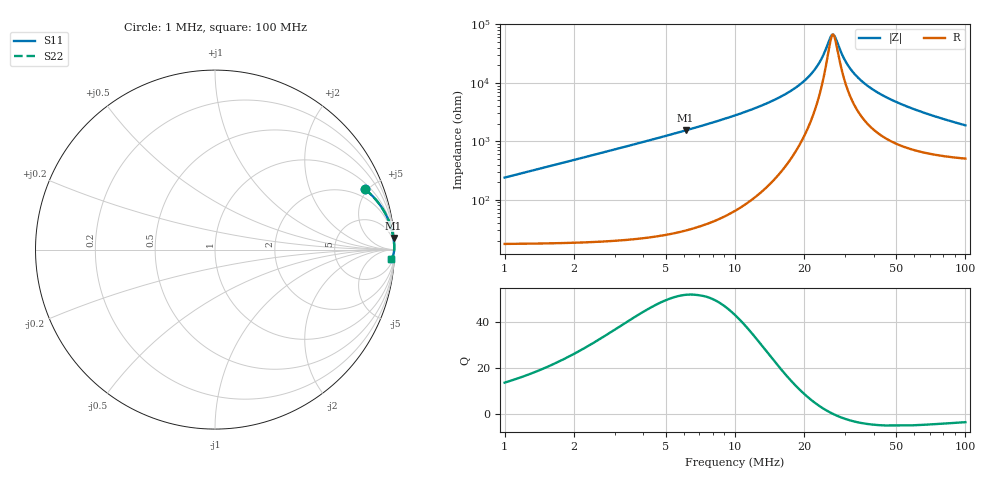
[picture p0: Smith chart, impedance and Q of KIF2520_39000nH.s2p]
!version-2
!date-12.2020
!Series
# MHz S RI R 50
!Freq ReS11 ImS11 ReS21 ImS21 ReS12 ImS12 ReS22 ImS22
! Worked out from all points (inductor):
!   991 points, 1 MHz to 100 MHz, reference 50 ohm
!   read as one part in series: L = 37.9 uH near 1.4 MHz
!   highest Q = 51.7 at 6.1 MHz (marker M1), where L = 40 uH
!   self-resonance near 26.6 MHz
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1  0.8339 0.3373  0.1661 -0.3373  0.1661 -0.3373  0.8339 0.3373
1.9  0.9465 0.2058  0.0535 -0.2058  0.0535 -0.2058  0.9465 0.2058
3.1  0.9792 0.1302  0.0208 -0.1302  0.0208 -0.1302  0.9792 0.1302
4.4  0.9896 0.0916  0.0104 -0.0916  0.0104 -0.0916  0.9896 0.0916
6.1  0.9945 0.0647  0.00547 -0.0647  0.00547 -0.0647  0.9945 0.0647
9.3  0.9976 0.0395  0.00242 -0.0395  0.00242 -0.0395  0.9976 0.0395
17.5  0.9989 0.0136  0.00112 -0.0136  0.00112 -0.0136  0.9989 0.0136
20.3  0.9989 0.00864  0.00115 -0.00864  0.00115 -0.00864  0.9989 0.00864
22.4  0.9988 0.00548  0.00122 -0.00548  0.00122 -0.00548  0.9988 0.00548
24  0.9987 0.00329  0.00131 -0.00329  0.00131 -0.00329  0.9987 0.00329
25.9  0.9986 0.000905  0.00143 -0.000905  0.00143 -0.000905  0.9986 0.000905
26.5  0.9985 0.000189  0.00147 -0.000189  0.00147 -0.000189  0.9985 0.000189
27.2  0.9985 -0.000624  0.00153 0.000624  0.00153 0.000624  0.9985 -0.000624
29  0.9983 -0.00263  0.00168 0.00263  0.00168 0.00263  0.9983 -0.00263
30.4  0.9982 -0.0041  0.00181 0.0041  0.00181 0.0041  0.9982 -0.0041
34  0.9978 -0.00763  0.00218 0.00763  0.00218 0.00763  0.9978 -0.00763
37  0.9975 -0.0103  0.00254 0.0103  0.00254 0.0103  0.9975 -0.0103
40.7  0.997 -0.0135  0.00303 0.0135  0.00303 0.0135  0.997 -0.0135
50.5  0.9954 -0.0209  0.00457 0.0209  0.00457 0.0209  0.9954 -0.0209
67  0.9921 -0.0318  0.00788 0.0318  0.00788 0.0318  0.9921 -0.0318
83.5  0.9881 -0.0413  0.0119 0.0413  0.0119 0.0413  0.9881 -0.0413
100  0.9833 -0.0497  0.0167 0.0497  0.0167 0.0497  0.9833 -0.0497
